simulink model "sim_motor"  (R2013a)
settings: Solver=ode4  StartTime=0.0  StopTime=t_stop  FixedStep=Ts  MaxStep=1e-3  RelTol=1e-3
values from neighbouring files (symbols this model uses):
  i_max = 70    [parameter_tracking.m]
  noise_psd_i = (sigma_noise_1/2)^2*Ts    (= 0.00049)    [parameter_tracking.m]
  noise_psd_w = (sigma_noise_2/2)^2*Ts    (= 0.001)    [parameter_tracking.m]
  p_ident = zeros(num_of_D,1)    [parameter_tracking.m]
  p_plant = p_plant_new    [parameter_tracking.m]
  penalty_factor = 0.1    [parameter_tracking.m]
  rand_seed_1 = round(rand*2^32)    [parameter_tracking.m]
  rand_seed_2 = round(rand*2^32)    [parameter_tracking.m]
  rand_seed_3 = round(rand*2^32)    [parameter_tracking.m]
  torque_step_time = 0.5    [parameter_tracking.m]
  Ts = 0.001    [parameter_tracking.m]
  w_max = 100    [parameter_tracking.m]
libraries: simulink x3

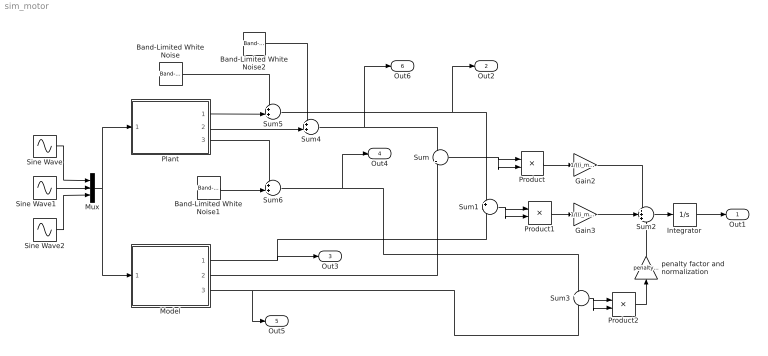
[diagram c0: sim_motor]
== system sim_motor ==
  Band-Limited White Noise : simulink/Sources/Band-Limited White Noise  Cov=[noise_psd_i]  Ts=Ts  seed=[rand_seed_1]
  Band-Limited White Noise1 : simulink/Sources/Band-Limited White Noise  Cov=[noise_psd_w]  Ts=Ts  seed=[rand_seed_3]
  Band-Limited White Noise2 : simulink/Sources/Band-Limited White Noise  Cov=[noise_psd_i]  Ts=Ts  seed=[rand_seed_2]
  Gain2 : Gain  Gain=1/((i_max)^2)
  Gain3 : Gain  Gain=1/((i_max)^2)
  Integrator : Integrator
  Model : Subsystem
  Mux : Mux  Inputs=3
  Plant : Subsystem
  Product : Product
  Product1 : Product
  Product2 : Product
  Sine Wave : Sin  Amplitude=325  Frequency=2*pi*50  SampleTime=0
  Sine Wave1 : Sin  Amplitude=325  Frequency=2*pi*50  Phase=-2*pi/3  SampleTime=0
  Sine Wave2 : Sin  Amplitude=325  Frequency=2*pi*50  Phase=2*pi/3  SampleTime=0
  Sum : Sum  Inputs=+|-
  Sum1 : Sum  Inputs=+|-
  Sum2 : Sum  Inputs=+++
  Sum3 : Sum  Inputs=+|-
  Sum4 : Sum  Inputs=++|
  Sum5 : Sum  Inputs=++|
  Sum6 : Sum  Inputs=++|
  penalty factor and normalization : Gain  Gain=penalty_factor/(w_max^2)
  Out1 : Outport
  Out2 : Outport  Port=2
  Out3 : Outport  Port=3
  Out4 : Outport  Port=4
  Out5 : Outport  Port=5
  Out6 : Outport  Port=6
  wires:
  Sine Wave/1 -> Mux/1
  Sine Wave2/1 -> Mux/3
  Sine Wave1/1 -> Mux/2
  Mux/1 -> Plant/1(uabc), Model/1(uabc)
  Model/2(is_beta) -> Sum/2
  Model/1(is_alfa) -> Sum1/2, Out3/1
  Sum/1 -> Product/2, Product/1
  Sum1/1 -> Product1/2, Product1/1
  Product/1 -> Gain2/1
  Sum2/1 -> Integrator/1
  Integrator/1 -> Out1/1
  Model/3(w) -> Out5/1, Sum3/2
  Product1/1 -> Gain3/1
  Sum5/1 -> Sum1/1, Out2/1
  Plant/1(is_alfa) -> Sum5/2
  Sum4/1 -> Sum/1, Out6/1
  Band-Limited White Noise/1 -> Sum5/1
  Plant/2(is_beta) -> Sum4/2
  Sum6/1 -> Out4/1, Sum3/1
  Band-Limited White Noise1/1 -> Sum6/2
  Plant/3(w) -> Sum6/1
  Sum3/1 -> Product2/2, Product2/1
  Product2/1 -> penalty factor and normalization/1
  penalty factor and normalization/1 -> Sum2/3
  Gain2/1 -> Sum2/1
  Gain3/1 -> Sum2/2
  Band-Limited White Noise2/1 -> Sum4/1

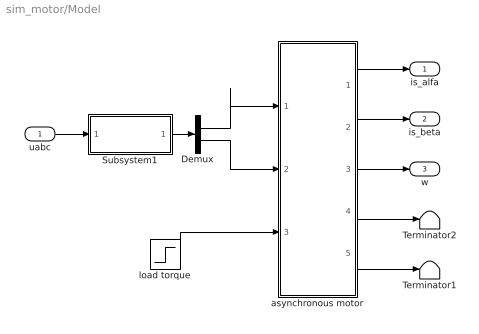
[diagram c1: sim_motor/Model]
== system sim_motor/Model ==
  uabc : Inport
  Demux : Demux  Outputs=2
  Subsystem1 : Subsystem
  Terminator1 : Terminator
  Terminator2 : Terminator
  asynchronous motor : Subsystem
  load torque : Step  Time=torque_step_time  After=20  SampleTime=0
  is_alfa : Outport
  is_beta : Outport  Port=2
  w : Outport  Port=3
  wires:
  uabc/1 -> Subsystem1/1(abc)
  asynchronous motor/2(is beta) -> is_beta/1
  asynchronous motor/1(is alfa) -> is_alfa/1
  asynchronous motor/4(psi _sa) -> Terminator2/1
  asynchronous motor/5(psi_sb) -> Terminator1/1
  Demux/2 -> asynchronous motor/2(Us beta)
  Demux/1 -> asynchronous motor/1(Us alfa)
  Subsystem1/1(alfa beta) -> Demux/1
  load torque/1 -> asynchronous motor/3(T_load)
  asynchronous motor/3(speed) -> w/1

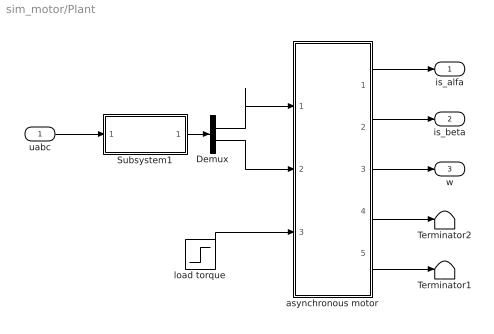
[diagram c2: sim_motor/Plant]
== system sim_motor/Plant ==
  uabc : Inport
  Demux : Demux  Outputs=2
  Subsystem1 : Subsystem
  Terminator1 : Terminator
  Terminator2 : Terminator
  asynchronous motor : Subsystem
  load torque : Step  Time=torque_step_time  After=20  SampleTime=0
  is_alfa : Outport
  is_beta : Outport  Port=2
  w : Outport  Port=3
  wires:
  asynchronous motor/3(speed) -> w/1
  load torque/1 -> asynchronous motor/3(T_load)
  Subsystem1/1(alfa beta) -> Demux/1
  Demux/1 -> asynchronous motor/1(Us alfa)
  Demux/2 -> asynchronous motor/2(Us beta)
  asynchronous motor/5(psi_sb) -> Terminator1/1
  asynchronous motor/4(psi _sa) -> Terminator2/1
  asynchronous motor/1(is alfa) -> is_alfa/1
  asynchronous motor/2(is beta) -> is_beta/1
  uabc/1 -> Subsystem1/1(abc)

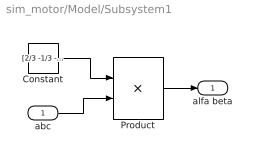
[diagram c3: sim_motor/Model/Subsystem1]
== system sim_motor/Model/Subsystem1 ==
  abc : Inport
  Constant : Constant  Value=[2/3 -1/3 -1/3;0 1/sqrt(3) -1/sqrt(3)]
  Product : Product  Multiplication=Matrix(*)
  alfa beta : Outport
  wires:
  Constant/1 -> Product/1
  abc/1 -> Product/2
  Product/1 -> alfa beta/1

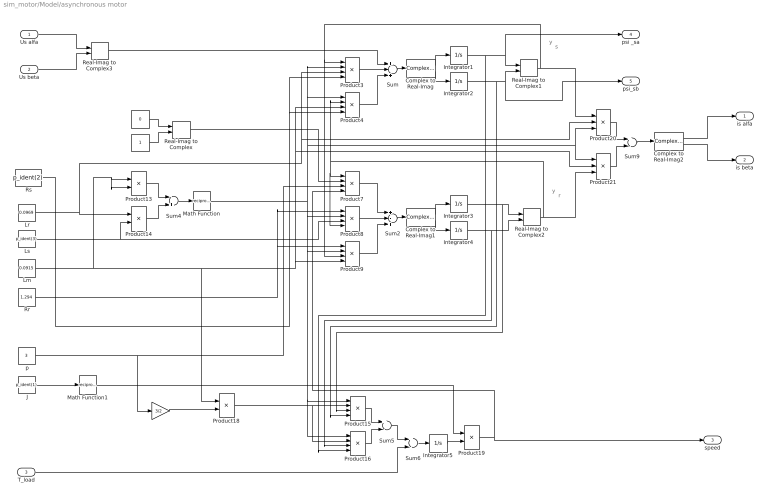
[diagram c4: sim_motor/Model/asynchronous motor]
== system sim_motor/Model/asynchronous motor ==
  note: r
  note: y
  note: s
  note: y
  Us alfa : Inport
  Us beta : Inport  Port=2
  T_load : Inport  Port=3
  " " : Constant  Value=0
  "  " : Constant
  "   " : Gain  Gain=3/2
  " J" : Constant  Value=p_ident(1)
  " Lm" : Constant  Value=0.0915
  " Lr" : Constant  Value=0.0969
  " Ls" : Constant  Value=p_ident(3)
  " Rr" : Constant  Value=1.294
  " Rs" : Constant  Value=p_ident(2)
  " p" : Constant  Value=3
  Complex to Real-Imag : ComplexToRealImag
  Complex to Real-Imag1 : ComplexToRealImag
  Complex to Real-Imag2 : ComplexToRealImag
  Integrator{1..5} (5 alike) : Integrator
  Math Function : Math  Operator=reciprocal
  Math Function1 : Math  Operator=reciprocal
  Product{13..14,18..19} (4 alike) : Product
  Product{3..4,7..9,15..16} (7 alike) : Product  Inputs=4
  Product20 : Product  Inputs=3
  Product21 : Product  Inputs=3
  Real-Imag to Complex{,1..3} (4 alike) : RealImagToComplex
  Sum : Sum  Inputs=+-+
  Sum2 : Sum  Inputs=+-+
  Sum4 : Sum  Inputs=-+
  Sum5 : Sum  Inputs=+-
  Sum6 : Sum  Inputs=+-
  Sum9 : Sum  Inputs=+-
  is alfa : Outport
  is beta : Outport  Port=2
  speed : Outport  Port=3
  psi _sa : Outport  Port=4
  psi_sb : Outport  Port=5
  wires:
  Product19/1 -> Product7/4, speed/1
  Complex to Real-Imag2/2 -> is beta/1
  Complex to Real-Imag2/1 -> is alfa/1
  " Rs"/1 -> Product4/4, Product3/4
  Real-Imag to Complex3/1 -> Sum/1
  Sum9/1 -> Complex to Real-Imag2/1
  Us alfa/1 -> Real-Imag to Complex3/1
  Us beta/1 -> Real-Imag to Complex3/2
  Product21/1 -> Sum9/2
  Product20/1 -> Sum9/1
  Real-Imag to Complex2/1 -> Product21/3, Product8/4, Product7/1, Product4/2
  Real-Imag to Complex1/1 -> Product20/1, Product9/3, Product3/1
  Sum5/1 -> Sum6/1
  " Ls"/1 -> Product8/3, Product14/2
  Integrator1/1 -> psi _sa/1, Real-Imag to Complex1/1, Product16/4
  Integrator4/1 -> Real-Imag to Complex2/2, Product16/3
  Integrator2/1 -> psi_sb/1, Real-Imag to Complex1/2, Product15/4
  Integrator3/1 -> Real-Imag to Complex2/1, Product15/3
  " Rr"/1 -> Product8/1, Product9/1
  Math Function/1 -> Product21/1, Product20/3, Product4/1, Product3/2, Product16/1, Product15/1, Product9/2, Product8/2
  Complex to Real-Imag1/2 -> Integrator4/1
  Complex to Real-Imag1/1 -> Integrator3/1
  Sum2/1 -> Complex to Real-Imag1/1
  Product9/1 -> Sum2/3
  Product8/1 -> Sum2/2
  Product7/1 -> Sum2/1
  Real-Imag to Complex/1 -> Product7/2
  Math Function1/1 -> Product19/1
  Integrator5/1 -> Product19/2
  T_load/1 -> Sum6/2
  Product16/1 -> Sum5/2
  Product15/1 -> Sum5/1
  Sum6/1 -> Integrator5/1
  Complex to Real-Imag/2 -> Integrator2/1
  Complex to Real-Imag/1 -> Integrator1/1
  Sum/1 -> Complex to Real-Imag/1
  Product3/1 -> Sum/2
  Product4/1 -> Sum/3
  "   "/1 -> Product18/2
  Product18/1 -> Product16/2, Product15/2
  " p"/1 -> "   "/1, Product7/3
  " J"/1 -> Math Function1/1
  "  "/1 -> Real-Imag to Complex/2
  " "/1 -> Real-Imag to Complex/1
  Sum4/1 -> Math Function/1
  Product14/1 -> Sum4/2
  Product13/1 -> Sum4/1
  " Lm"/1 -> Product21/2, Product4/3, Product9/4, Product18/1, Product13/2, Product13/1
  " Lr"/1 -> Product20/2, Product3/3, Product14/1

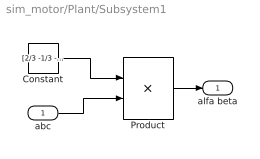
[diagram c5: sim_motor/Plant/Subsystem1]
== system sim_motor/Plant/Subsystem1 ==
  abc : Inport
  Constant : Constant  Value=[2/3 -1/3 -1/3;0 1/sqrt(3) -1/sqrt(3)]
  Product : Product  Multiplication=Matrix(*)
  alfa beta : Outport
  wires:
  Product/1 -> alfa beta/1
  abc/1 -> Product/2
  Constant/1 -> Product/1

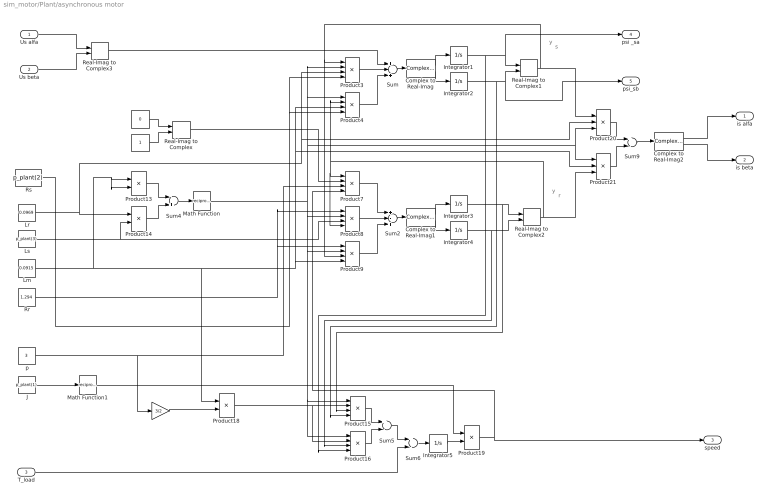
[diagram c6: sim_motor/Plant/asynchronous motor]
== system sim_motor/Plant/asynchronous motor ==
  note: y
  note: s
  note: y
  note: r
  Us alfa : Inport
  Us beta : Inport  Port=2
  T_load : Inport  Port=3
  " " : Constant  Value=0
  "  " : Constant
  "   " : Gain  Gain=3/2
  " J" : Constant  Value=p_plant(1)
  " Lm" : Constant  Value=0.0915
  " Lr" : Constant  Value=0.0969
  " Ls" : Constant  Value=p_plant(3)
  " Rr" : Constant  Value=1.294
  " Rs" : Constant  Value=p_plant(2)
  " p" : Constant  Value=3
  Complex to Real-Imag : ComplexToRealImag
  Complex to Real-Imag1 : ComplexToRealImag
  Complex to Real-Imag2 : ComplexToRealImag
  Integrator{1..5} (5 alike) : Integrator
  Math Function : Math  Operator=reciprocal
  Math Function1 : Math  Operator=reciprocal
  Product{13..14,18..19} (4 alike) : Product
  Product{3..4,7..9,15..16} (7 alike) : Product  Inputs=4
  Product20 : Product  Inputs=3
  Product21 : Product  Inputs=3
  Real-Imag to Complex{,1..3} (4 alike) : RealImagToComplex
  Sum : Sum  Inputs=+-+
  Sum2 : Sum  Inputs=+-+
  Sum4 : Sum  Inputs=-+
  Sum5 : Sum  Inputs=+-
  Sum6 : Sum  Inputs=+-
  Sum9 : Sum  Inputs=+-
  is alfa : Outport
  is beta : Outport  Port=2
  speed : Outport  Port=3
  psi _sa : Outport  Port=4
  psi_sb : Outport  Port=5
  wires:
  " Lr"/1 -> Product14/1, Product3/3, Product20/2
  " Lm"/1 -> Product13/1, Product13/2, Product18/1, Product9/4, Product4/3, Product21/2
  Product13/1 -> Sum4/1
  Product14/1 -> Sum4/2
  Sum4/1 -> Math Function/1
  " "/1 -> Real-Imag to Complex/1
  "  "/1 -> Real-Imag to Complex/2
  " J"/1 -> Math Function1/1
  " p"/1 -> Product7/3, "   "/1
  Product18/1 -> Product15/2, Product16/2
  "   "/1 -> Product18/2
  Product4/1 -> Sum/3
  Product3/1 -> Sum/2
  Sum/1 -> Complex to Real-Imag/1
  Complex to Real-Imag/1 -> Integrator1/1
  Complex to Real-Imag/2 -> Integrator2/1
  Sum6/1 -> Integrator5/1
  Product15/1 -> Sum5/1
  Product16/1 -> Sum5/2
  T_load/1 -> Sum6/2
  Integrator5/1 -> Product19/2
  Math Function1/1 -> Product19/1
  Real-Imag to Complex/1 -> Product7/2
  Product7/1 -> Sum2/1
  Product8/1 -> Sum2/2
  Product9/1 -> Sum2/3
  Sum2/1 -> Complex to Real-Imag1/1
  Complex to Real-Imag1/1 -> Integrator3/1
  Complex to Real-Imag1/2 -> Integrator4/1
  Math Function/1 -> Product8/2, Product9/2, Product15/1, Product16/1, Product3/2, Product4/1, Product20/3, Product21/1
  " Rr"/1 -> Product9/1, Product8/1
  Integrator3/1 -> Product15/3, Real-Imag to Complex2/1
  Integrator2/1 -> Product15/4, Real-Imag to Complex1/2, psi_sb/1
  Integrator4/1 -> Product16/3, Real-Imag to Complex2/2
  Integrator1/1 -> Product16/4, Real-Imag to Complex1/1, psi _sa/1
  " Ls"/1 -> Product14/2, Product8/3
  Sum5/1 -> Sum6/1
  Real-Imag to Complex1/1 -> Product3/1, Product9/3, Product20/1
  Real-Imag to Complex2/1 -> Product4/2, Product7/1, Product8/4, Product21/3
  Product20/1 -> Sum9/1
  Product21/1 -> Sum9/2
  Us beta/1 -> Real-Imag to Complex3/2
  Us alfa/1 -> Real-Imag to Complex3/1
  Sum9/1 -> Complex to Real-Imag2/1
  Real-Imag to Complex3/1 -> Sum/1
  " Rs"/1 -> Product3/4, Product4/4
  Complex to Real-Imag2/1 -> is alfa/1
  Complex to Real-Imag2/2 -> is beta/1
  Product19/1 -> Product7/4, speed/1
